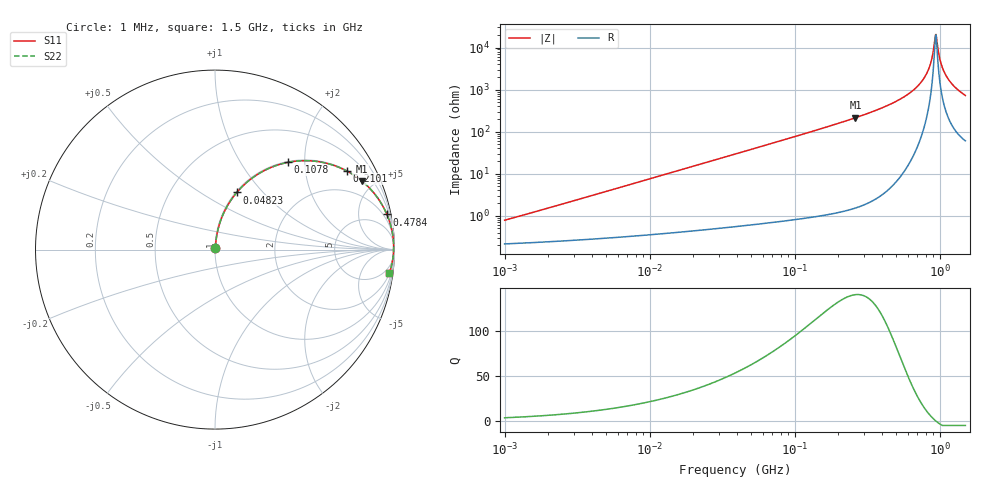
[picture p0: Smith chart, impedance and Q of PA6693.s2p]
# MHz S MA R 50
!Freq  MagS11  AngS11  MagS21  AngS21  MagS12  AngS12  MagS22  AngS22
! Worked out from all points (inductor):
!   801 points, 1 MHz to 1.5 GHz, reference 50 ohm
!   read as one part in series: L = 120 nH near 1.037 MHz
!   highest Q = 140 at 261.7 MHz (marker M1), where L = 130 nH
!   self-resonance near 932.5 MHz
!   S11 on the Smith chart (normalised r, x): 1 MHz: 1.00, +0.02; 48.23 MHz: 1.01, +0.73; 107.8 MHz: 1.02, +1.65; 210.1 MHz: 1.02, +3.34; 478.4 MHz: 1.11, +9.75; 1.5 GHz: 2, -14
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1  0.007821 73.7  0.9978 -0.4  0.9978 -0.4  0.007821 73.7
3.404045  0.02573 82.6  0.997 -1.5  0.997 -1.5  0.02573 82.6
11.48208  0.08603 82.6  0.9927 -4.9  0.9927 -4.9  0.08603 82.6
38.72983  0.2794 72.7  0.9549 -16.2  0.9549 -16.2  0.2794 72.7
48.23123  0.3408 69.1  0.9346 -19.9  0.9346 -19.9  0.3408 69.1
107.8198  0.6327 50.2  0.768 -39.2  0.768 -39.2  0.6327 50.2
131.8381  0.7088 44.3  0.699 -45.1  0.699 -45.1  0.7088 44.3
210.1439  0.8549 30.8  0.5125 -58.7  0.5125 -58.7  0.8549 30.8
261.6974  0.9035 25.0  0.4222 -64.6  0.4222 -64.6  0.9035 25.0
444.6989  0.9722 13.0  0.2248 -76.4  0.2248 -76.4  0.9722 13.0
478.4395  0.9775 11.6  0.2005 -77.8  0.2005 -77.8  0.9775 11.6
635.1854  0.991 6.4  0.1121 -82.2  0.1121 -82.2  0.991 6.4
762.6106  0.9948 3.4  0.05878 -83.3  0.05878 -83.3  0.9948 3.4
843.2844  0.9955 1.7  0.03034 -80.7  0.03034 -80.7  0.9955 1.7
874.6907  0.9956 1.1  0.0202 -76.7  0.0202 -76.7  0.9956 1.1
915.5986  0.9954 0.4  0.008263 -56.0  0.008263 -56.0  0.9954 0.4
941.0559  0.9952 -0.0  0.004864 9.8  0.004864 9.8  0.9952 -0.0
967.2211  0.9949 -0.5  0.009906 59.0  0.009906 59.0  0.9949 -0.5
1031.138  0.994 -1.5  0.02712 76.5  0.02712 76.5  0.994 -1.5
1109.373  0.9925 -2.7  0.04759 79.6  0.04759 79.6  0.9925 -2.7
1260.837  0.9884 -4.8  0.08401 79.7  0.08401 79.7  0.9884 -4.8
1500  0.9797 -7.7  0.1349 77.5  0.1349 77.5  0.9797 -7.7
